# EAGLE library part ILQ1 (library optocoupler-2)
SIEMENS OPTO COUPLER
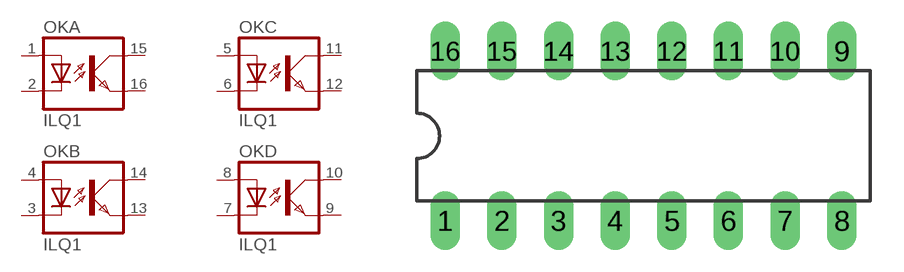
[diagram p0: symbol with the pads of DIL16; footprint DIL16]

Designator prefix OK; gates A=OK B=OK C=OK D=OK

## ILQ1  [DIL16]
1  A:A  pas
2  A:C  pas
3  B:C  pas
4  B:A  pas
5  C:A  pas
6  C:C  pas
7  D:C  pas
8  D:A  pas
9  D:EMIT  pas
10  D:COL  pas
11  C:COL  pas
12  C:EMIT  pas
13  B:EMIT  pas
14  B:COL  pas
15  A:COL  pas
16  A:EMIT  pas

## Footprint DIL16 (pad centres in mm)
Dual In Line Package
drill 0.813 long: 1 -8.89,-3.81; 2 -6.35,-3.81; 3 -3.81,-3.81; 4 -1.27,-3.81; 5 1.27,-3.81; 6 3.81,-3.81; 7 6.35,-3.81; 8 8.89,-3.81; 9 8.89,3.81; 10 6.35,3.81; 11 3.81,3.81; 12 1.27,3.81; 13 -1.27,3.81; 14 -3.81,3.81; 15 -6.35,3.81; 16 -8.89,3.81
